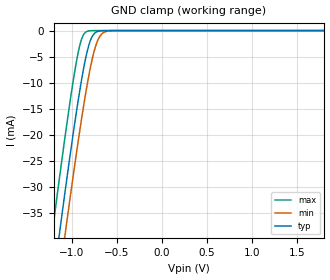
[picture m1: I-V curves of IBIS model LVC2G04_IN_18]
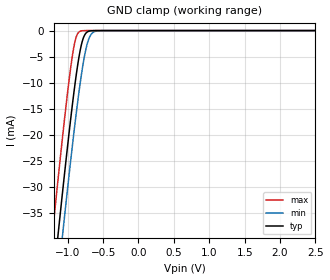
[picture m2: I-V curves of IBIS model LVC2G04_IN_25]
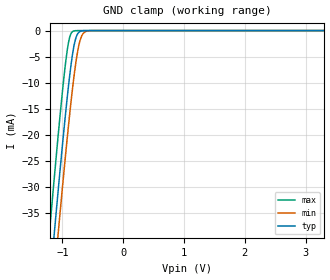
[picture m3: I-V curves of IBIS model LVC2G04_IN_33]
| TEXAS INSTRUMENTS INCORPORATED
| Standard Linear and Logic Group
| IBIS Model of SN74LVC2G04
| DUAL INVERTER GATE
| This file contains package information for the following:
|  SOT 6-pin (DCK) package as [Component] LVC2G04_DCK
|  SOT 6-pin (DBV) package as [Component] LVC2G04_DBV
|  DSBGA 6-pin (YEA) package as [Component] LVC2G04_YEA
|  DSBGA 6-pin (YZA) package as [Component] LVC2G04_YZA
|  DSBGA 6-pin (YEP) package as [Component] LVC2G04_YEP
|  DSBGA 6-pin (YZP) package as [Component] LVC2G04_YZP
| This device can be powered at the following Vccs:
|  1.8 volt Vcc
|  2.5 volt Vcc
|  3.3 volt Vcc
|  5 volt Vcc
| This file provides unique models under the [Model Selector] for each Vcc.
| For operation at a specific Vcc, select the appropriate model after each
| [Model Selector] keyword.
[IBIS Ver]   3.2
[Comment char]  |_char
[File Name]   sn74lvc2g04.ibs
[File Rev]   1.1 | d_die
[Date]   July 15, 2004
[Source]   Data created from TI-SPICE simulations at TI-SLL.
[Notes]   The following is an IBIS list for the SN74LVC2G04.
   Please contact sllibis@ti.com with questions and
   comments concerning SLL IBIS models.
   - FILE REV HISTORY
   - 1.1 Release IBIS file on 04/26/02
   - 1.2 YEP and YZP packages added 07/15/04
   - Due to the fact that the device is 5-V input/output
   tolerant, the output model has some non-monotonic
   warnings.
[Disclaimer] Property of Texas Instruments Incorporated.  Unauthorized
   reproduction and/or distribution is strictly prohibited.
   This product is protected under copyright law.
   Created  2002, (C) Copyright  2002, Texas Instruments
   Incorporated, All Rights Reserved
   UNLESS THERE IS A SIGNED, WRITTEN AGREEMENT TO THE
   CONTRARY, TEXAS INSTRUMENTS (TI) IS PROVIDING THE IBIS
   MODELS  AND WITHOUT ANY WARRANTY, EXPRESSED OR
   IMPLIED.  TI assumes no liability for:
   1) the accuracy of the IBIS models provided to your
   company;
   2) the proper functioning of these IBIS Models in your
   design or for any resulting applications; or
   3) infringement of patents, copyrights or intellectual
   property rights resulting from your use of these IBIS
   models.
   TI provides IBIS Models as a service to our customers.
   You and your company shall not distribute, sell or give
   these models to anyone else without prior written
   permission from TI.
   TI reserves the right to make changes to our products or
   to discontinue any semiconductor product or service
   without notice, and advises our customers to obtain the
   latest version of relevant information to verify, before
   placing orders, that the information being relied on is
   current.
   Please be aware that your receipt and use of the IBIS
   information provided shall serve as acceptance of these
   terms and conditions. If you do not accept these terms,
   you should return or destroy the IBIS models and any
   other accompanying information immediately.
| Component LVC2G04_DCK 6-pin SOT
[Component]   LVC2G04_DCK
[Manufacturer]   Texas Instruments, Inc.
[Package]
|   typ   min   max
R_pkg   1.400e-02   1.100e-02   2.100e-02
L_pkg   9.480e-10   7.840e-10   1.103e-09
C_pkg   1.910e-13   1.670e-13   2.050e-13
[Pin]   signal_name   model_name   R_pin   L_pin   C_pin
1   1A   LVC2G04_IN   1.300e-02   9.840e-10   1.960e-13
2   GND   GND   2.100e-02   1.103e-09   2.050e-13
3   2A   LVC2G04_IN   1.100e-02   9.980e-10   1.970e-13
4   2Y   LVC2G04_OUT   1.300e-02   9.040e-10   1.900e-13
5   VCC   POWER   1.500e-02   7.840e-10   1.670e-13
6   1Y   LVC2G04_OUT   1.200e-02   9.160e-10   1.950e-13
| Component LVC2G04_DBV 6-pin SOT
[Component]   LVC2G04_DBV
[Manufacturer]   Texas Instruments, Inc.
[Package]
|   typ   min   max
R_pkg   0.025   0.019   0.037
L_pkg   1.524nH   1.260nH   1.751nH
C_pkg   0.245pF   0.198pF   0.264pF
[Pin]   signal_name   model_name   R_pin   L_pin   C_pin
1   1A   LVC2G04_IN   0.021   1.405nH   0.246pF
2   GND   GND   0.037   1.751nH   0.263pF
3   2A   LVC2G04_IN   0.026   1.493nH   0.247pF
4   2Y   LVC2G04_OUT   0.019   1.620nH   0.264pF
5   VCC   POWER   0.024   1.260nH   0.198pF
6   1Y   LVC2G04_OUT   0.021   1.617nH   0.250pF
| Component LVC2G04_YEA 6-pin NanoStar WCSP
[Component]   LVC2G04_YEA
[Manufacturer]   Texas Instruments, Inc.
[Package]
|   typ   min   max
R_pkg   0.001   0.001   0.001
L_pkg   1.021nH   1.021nH   1.021nH
C_pkg   0.047pF   0.046pF   0.047pF
[Pin]   signal_name   model_name   R_pin   L_pin   C_pin
1   1A   LVC2G04_IN   0.001   0.021nH   0.046pF
2   GND   GND   0.001   0.021nH   0.047pF
3   2A   LVC2G04_IN   0.001   0.021nH   0.046pF
4   2Y   LVC2G04_OUT   0.001   0.021nH   0.046pF
5   VCC   POWER   0.001   0.021nH   0.047pF
6   1Y   LVC2G04_OUT   0.001   0.021nH   0.046pF
| Component LVC2G04_YZA 6-pin NanoFree WCSP
[Component]   LVC2G04_YZA
[Manufacturer]   Texas Instruments, Inc.
[Package]
|   typ   min   max
R_pkg   0.001   0.001   0.001
L_pkg   1.021nH   1.021nH   1.021nH
C_pkg   0.047pF   0.046pF   0.047pF
[Pin]   signal_name   model_name   R_pin   L_pin   C_pin
1   1A   LVC2G04_IN   0.001   0.021nH   0.046pF
2   GND   GND   0.001   0.021nH   0.047pF
3   2A   LVC2G04_IN   0.001   0.021nH   0.046pF
4   2Y   LVC2G04_OUT   0.001   0.021nH   0.046pF
5   VCC   POWER   0.001   0.021nH   0.047pF
6   1Y   LVC2G04_OUT   0.001   0.021nH   0.046pF
| Component LVC2G04_YEP 6-pin DSBGA
[Component]   LVC2G04_YEP
[Manufacturer]   Texas Instruments, Inc.
[Package]
|   typ   min   max
R_pkg   1.000e-03   1.000e-03   1.000e-03
L_pkg   2.460e-11   2.400e-11   2.500e-11
C_pkg   6.500e-14   6.400e-14   6.700e-14
[Pin]   signal_name   model_name   R_pin   L_pin   C_pin
1   1A   LVC2G04_IN   1.000e-03   2.500e-11   6.400e-14
2   GND   GND   1.000e-03   2.400e-11   6.700e-14
3   2A   LVC2G04_IN   1.000e-03   2.500e-11   6.400e-14
4   2Y   LVC2G04_OUT   1.000e-03   2.500e-11   6.400e-14
5   VCC   POWER   1.000e-03   2.400e-11   6.700e-14
6   1Y   LVC2G04_OUT   1.000e-03   2.500e-11   6.400e-14
| Component LVC2G04_YZP 6-pin DSBGA
[Component]   LVC2G04_YZP
[Manufacturer]   Texas Instruments, Inc.
[Package]
|   typ   min   max
R_pkg   1.000e-03   1.000e-03   1.000e-03
L_pkg   2.460e-11   2.400e-11   2.500e-11
C_pkg   6.500e-14   6.400e-14   6.700e-14
[Pin]   signal_name   model_name   R_pin   L_pin   C_pin
1   1A   LVC2G04_IN   1.000e-03   2.500e-11   6.400e-14
2   GND   GND   1.000e-03   2.400e-11   6.700e-14
3   2A   LVC2G04_IN   1.000e-03   2.500e-11   6.400e-14
4   2Y   LVC2G04_OUT   1.000e-03   2.500e-11   6.400e-14
5   VCC   POWER   1.000e-03   2.400e-11   6.700e-14
6   1Y   LVC2G04_OUT   1.000e-03   2.500e-11   6.400e-14
| Model LVC2G04_IN
[Model Selector]   LVC2G04_IN
LVC2G04_IN_18   1.8 volt Vcc
LVC2G04_IN_25   2.5 volt Vcc
LVC2G04_IN_33   3.3 volt Vcc
LVC2G04_IN_50   5 volt Vcc
| Model LVC2G04_OUT
[Model Selector]   LVC2G04_OUT
LVC2G04_OUT_18   1.8 volt Vcc
LVC2G04_OUT_25   2.5 volt Vcc
LVC2G04_OUT_33   3.3 volt Vcc
LVC2G04_OUT_50   5 volt Vcc
| Models and submodels in the file (8): LVC2G04_IN_18 (Input), LVC2G04_IN_25 (Input), LVC2G04_IN_33 (Input), LVC2G04_IN_50 (Input), LVC2G04_OUT_18 (Output), LVC2G04_OUT_25 (Output), LVC2G04_OUT_33 (Output), LVC2G04_OUT_50 (Output)
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[Model]   LVC2G04_IN_18
Model_type  Input
Vinl=0.5775
Vinh=1.2675
| variable   typ   min   max
C_comp   3.49pF   3.03pF   4.27pF
[Temperature Range]   40   100   -40
| Ambient temperature   25   85   -40
[Voltage range]   1.8   1.65   1.95
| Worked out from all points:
|   GND clamp passes 1 mA (typ) near -0.77 V on its own axis
[GND Clamp]
| LVC2G04_IN_18
|   Voltage   I(typ)   I(min)   I(max)
-5.5V     -655.2mA   -662.2mA   -646.6mA
-1.215V   -49.6mA    -57.88mA   -38.96mA
-1.135V   -39.07mA   -47.36mA   -28.42mA
-1.075V   -31.35mA   -39.6mA    -20.75mA
-1.055V   -28.82mA   -37.05mA   -18.27mA
-955mV    -16.68mA   -24.66mA   -6.874mA
-885mV    -9.098mA   -16.55mA   -1.486mA
-825mV    -3.922mA   -10.26mA   -137.1uA
-780mV    -1.472mA   -6.227mA   -17.15uA
-715mV    -205.4uA   -2.128mA   -808.5nA
-650mV    -22.01uA   -443.9uA   -37.93nA
1.8V      3.326pA    6.142pA    3.026pA
[Model]   LVC2G04_IN_25
Model_type  Input
Vinl=0.7
Vinh=1.7
| variable   typ   min   max
C_comp   3.42pF   2.82pF   4.35pF
[Temperature Range]   40   100   -40
| Ambient temperature   25   85   -40
[Voltage range]   2.5   2.3   2.7
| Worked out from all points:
|   GND clamp passes 1 mA (typ) near -0.77 V on its own axis
[GND Clamp]
| LVC2G04_IN_25
|   Voltage   I(typ)   I(min)   I(max)
-5.5V     -655.2mA   -662.2mA   -646.6mA
-1.215V   -49.6mA    -57.88mA   -38.96mA
-1.14V    -39.72mA   -48.01mA   -29.07mA
-1.12V    -37.12mA   -45.41mA   -26.48mA
-1.08V    -31.98mA   -40.25mA   -21.38mA
-1.06V    -29.44mA   -37.69mA   -18.89mA
-960mV    -17.26mA   -25.26mA   -7.377mA
-890mV    -9.597mA   -17.1mA    -1.734mA
-785mV    -1.671mA   -6.635mA   -21.67uA
-720mV    -242.5uA   -2.354mA   -1.023uA
-650mV    -22.01uA   -443.9uA   -37.93nA
2.5V      4.713pA    7.577pA    4.389pA
[Model]   LVC2G04_IN_33
Model_type  Input
Vinl=0.8
Vinh=2.0
| variable   typ   min   max
C_comp   3.34pF   2.67pF   4.38pF
[Temperature Range]   40   100   -40
| Ambient temperature   25   85   -40
[Voltage range]   3.3   3   3.6
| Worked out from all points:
|   GND clamp passes 1 mA (typ) near -0.77 V on its own axis
[GND Clamp]
| LVC2G04_IN_33
|   Voltage   I(typ)   I(min)   I(max)
-5.5V     -655.2mA   -662.2mA   -646.6mA
-1.225V   -50.93mA   -59.21mA   -40.3mA
-1.145V   -40.37mA   -48.66mA   -29.72mA
-1.12V    -37.12mA   -45.41mA   -26.48mA
-1.08V    -31.98mA   -40.25mA   -21.38mA
-1.06V    -29.44mA   -37.69mA   -18.89mA
-965mV    -17.84mA   -25.87mA   -7.89mA
-885mV    -9.098mA   -16.55mA   -1.486mA
-780mV    -1.472mA   -6.227mA   -17.15uA
-715mV    -205.4uA   -2.128mA   -808.5nA
-640mV    -15.53uA   -338.1uA   -23.69nA
3.3V      6.304pA    9.258pA    5.93pA
